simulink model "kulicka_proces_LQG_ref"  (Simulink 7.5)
libraries: mathlib x31, execlib x4, reglib x3, anallib x1, arclib x1

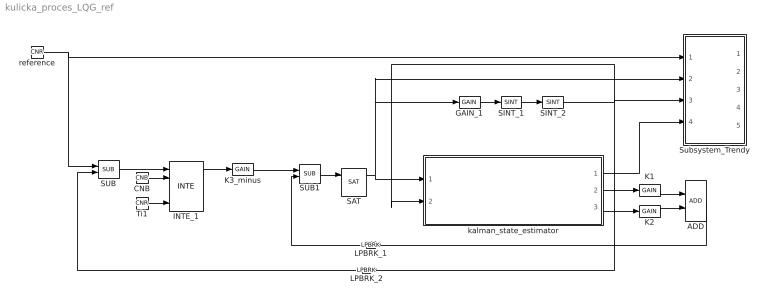
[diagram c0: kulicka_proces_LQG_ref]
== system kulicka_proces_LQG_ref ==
  ADD : mathlib/ADD  SystemSampleTime=-1
  CNB : mathlib/CNB  SystemSampleTime=-1  YCN=on
  GAIN_1 : mathlib/GAIN  SystemSampleTime=-1  k=7.14
  INTE_1 : anallib/INTE  ymin=-1  ymax=1
  K1 : mathlib/GAIN  SystemSampleTime=-1  k=0.2269
  K2 : mathlib/GAIN  SystemSampleTime=-1  k=0.1718
  K3_minus : mathlib/GAIN  SystemSampleTime=-1  k=0.057735
  LPBRK_1 : execlib/LPBRK  Orientation=left
  LPBRK_2 : execlib/LPBRK  Orientation=left
  SAT : reglib/SAT  SystemSampleTime=-1  tp=1  tn=1  hilim0=0.01  lolim0=-0.01  HLD=on
  SINT_1 : reglib/SINT  SystemSampleTime=-1  ti=1  y0=0  ymax=1000  ymin=-1000
  SINT_2 : reglib/SINT  SystemSampleTime=-1  ti=1  y0=0  ymax=1000  ymin=-1000
  SUB : mathlib/SUB  SystemSampleTime=-1
  SUB1 : mathlib/SUB  SystemSampleTime=-1
  Subsystem_Trendy : Subsystem
  Ti1 : mathlib/CNR  SystemSampleTime=-1  ycn=1
  kalman_state_estimator : Subsystem
  reference : mathlib/CNR  SystemSampleTime=-1  ycn=0.5
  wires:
  ADD/1 -> LPBRK_1/1
  CNB/1 -> INTE_1/2
  GAIN_1/1 -> SINT_1/1
  INTE_1/1 -> K3_minus/1
  K1/1 -> ADD/1
  K2/1 -> ADD/2
  K3_minus/1 -> SUB1/1
  LPBRK_1/1 -> SUB1/2
  LPBRK_2/1 -> SUB/2
  SAT/1 -> kalman_state_estimator/1(u), GAIN_1/1, Subsystem_Trendy/2(u_out)
  SINT_1/1 -> SINT_2/1
  SINT_2/1 -> LPBRK_2/1, Subsystem_Trendy/3(y_out), kalman_state_estimator/2(y)
  SUB/1 -> INTE_1/1
  SUB1/1 -> SAT/1
  Ti1/1 -> INTE_1/5
  kalman_state_estimator/1(y_kalman) -> Subsystem_Trendy/4(y_est)
  kalman_state_estimator/2(x1_kalman) -> K1/1
  kalman_state_estimator/3(x2_kalman) -> K2/1
  reference/1 -> SUB/1, Subsystem_Trendy/1(w_in)

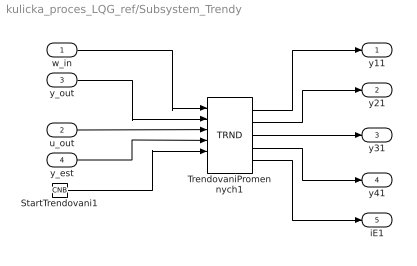
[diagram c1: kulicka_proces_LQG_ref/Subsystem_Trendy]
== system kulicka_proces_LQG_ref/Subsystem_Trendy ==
  w_in : Inport  Port=1
  u_out : Inport  Port=2
  y_out : Inport  Port=3
  y_est : Inport  Port=4
  StartTrendovani1 : mathlib/CNB  SystemSampleTime=-1  YCN=on
  TrendovaniPromennych1 : arclib/TRND  SystemSampleTime=-1  n=4  l=1000  btype=8: Double  ptype1=1: Store  ptype2=1: Store  ptype3=1: Store  ptype4=1: Store  pfac=1  afac=0  arc=2  id=1  Title=Trend Title
  y11 : Outport  Port=1
  y21 : Outport  Port=2
  y31 : Outport  Port=3
  y41 : Outport  Port=4
  iE1 : Outport  Port=5
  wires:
  StartTrendovani1/1 -> TrendovaniPromennych1/5
  TrendovaniPromennych1/1 -> y11/1
  TrendovaniPromennych1/2 -> y21/1
  TrendovaniPromennych1/3 -> y31/1
  TrendovaniPromennych1/4 -> y41/1
  TrendovaniPromennych1/5 -> iE1/1
  u_out/1 -> TrendovaniPromennych1/3
  w_in/1 -> TrendovaniPromennych1/1
  y_est/1 -> TrendovaniPromennych1/4
  y_out/1 -> TrendovaniPromennych1/2

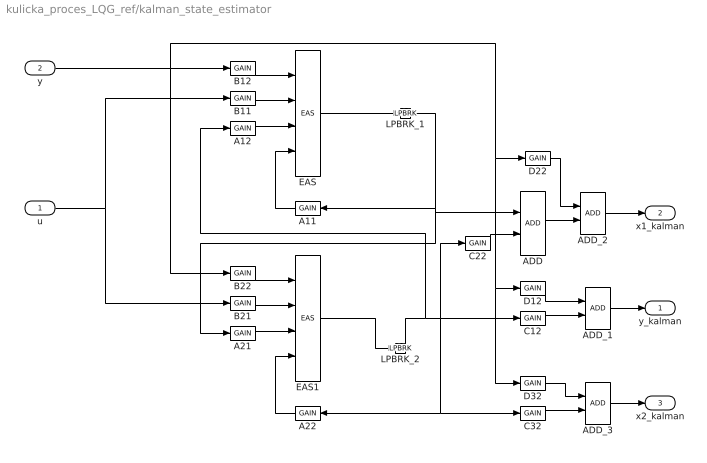
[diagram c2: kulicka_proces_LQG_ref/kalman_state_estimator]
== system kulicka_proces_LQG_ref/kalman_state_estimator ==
  u : Inport  Port=1
  y : Inport  Port=2
  A11 : mathlib/GAIN  Orientation=left  SystemSampleTime=-1  k=1
  A12 : mathlib/GAIN  SystemSampleTime=-1  k=-0.01972
  A21 : mathlib/GAIN  SystemSampleTime=-1  k=0.02
  A22 : mathlib/GAIN  Orientation=left  SystemSampleTime=-1  k=0.9717
  ADD : mathlib/ADD  SystemSampleTime=-1
  ADD_1 : mathlib/ADD  SystemSampleTime=-1
  ADD_2 : mathlib/ADD  SystemSampleTime=-1
  ADD_3 : mathlib/ADD  SystemSampleTime=-1
  B11 : mathlib/GAIN  SystemSampleTime=-1  k=0.1428
  B12 : mathlib/GAIN  SystemSampleTime=-1  k=0.01972
  B21 : mathlib/GAIN  SystemSampleTime=-1  k=0.001428
  B22 : mathlib/GAIN  SystemSampleTime=-1  k=0.02828
  C12 : mathlib/GAIN  SystemSampleTime=-1  k=0.9721
  C22 : mathlib/GAIN  SystemSampleTime=-1  k=-0.01972
  C32 : mathlib/GAIN  SystemSampleTime=-1  k=0.9721
  D12 : mathlib/GAIN  SystemSampleTime=-1  k=0.02789
  D22 : mathlib/GAIN  SystemSampleTime=-1  k=0.01972
  D32 : mathlib/GAIN  SystemSampleTime=-1  k=0.02789
  EAS : mathlib/EAS  SystemSampleTime=-1  a=1  b=1  c=1  d=1  y0=0
  EAS1 : mathlib/EAS  SystemSampleTime=-1  a=1  b=1  c=1  d=1  y0=0
  LPBRK_1 : execlib/LPBRK
  LPBRK_2 : execlib/LPBRK
  y_kalman : Outport  Port=1
  x1_kalman : Outport  Port=2
  x2_kalman : Outport  Port=3
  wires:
  A11/1 -> EAS/4
  A12/1 -> EAS/3
  A21/1 -> EAS1/3
  A22/1 -> EAS1/4
  ADD/1 -> ADD_2/2
  ADD_1/1 -> y_kalman/1
  ADD_2/1 -> x1_kalman/1
  ADD_3/1 -> x2_kalman/1
  B11/1 -> EAS/2
  B12/1 -> EAS/1
  B21/1 -> EAS1/2
  B22/1 -> EAS1/1
  C12/1 -> ADD_1/2
  C22/1 -> ADD/2
  C32/1 -> ADD_3/2
  D12/1 -> ADD_1/1
  D22/1 -> ADD_2/1
  D32/1 -> ADD_3/1
  EAS/1 -> LPBRK_1/1
  EAS1/1 -> LPBRK_2/1
  LPBRK_1/1 -> A11/1, A21/1, ADD/1
  LPBRK_2/1 -> A12/1, C12/1, C22/1, A22/1, C32/1
  u/1 -> B11/1, B21/1
  y/1 -> B12/1, B22/1, D22/1, D12/1, D32/1
